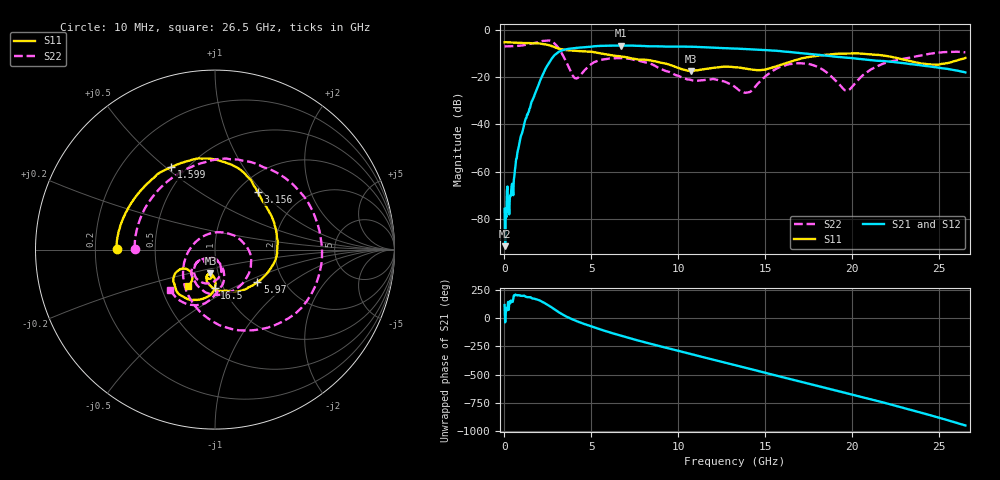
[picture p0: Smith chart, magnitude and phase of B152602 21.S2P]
!  2-Port S-parameters saved by WinCal
! VAR MeasName=S-Parameters (CALIBRATED_DATA) read from VNA (N5242A)
! VAR MeasDate=2016-1-5 16:28:22
! VAR NAME=B152602 21
! VAR FILENAME=B152602 21.S2P
! VAR DATE=2016-1-5 16:28:22
! VAR PHYS_PORTS=1,2
# Hz S DB R 50
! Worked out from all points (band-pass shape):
!   801 points, 10 MHz to 26.5 GHz, reference 50 ohm
!   highest |S21| = -6.62 dB at 6.699 GHz (marker M1); lowest = -91.6 dB at 43.11 MHz (marker M2)
!   |S21| within 3 dB of the highest: 3.062 GHz to 16.73 GHz (13.67 GHz wide, 138 % of centre)
!   lowest |S11| = -17.4 dB at 10.71 GHz (marker M3), VSWR 1.31, Z = 46 - j12.4 ohm
!   |S11| at or under -10 dB: 5.57 GHz to 19.66 GHz (14.09 GHz wide, 112 % of centre); 19.69 GHz to 19.82 GHz (129.6 MHz wide, 0.656 % of centre); 20.52 GHz to end of sweep
!   |S22| runs from -26.6 to -4.5 dB; largest |S21 - S12| = 0.0033
!   S11 on the Smith chart (normalised r, x): 10 MHz: 0.29, +0.00; 1.599 GHz: 0.41, +0.52; 3.156 GHz: 1.23, +0.94; 5.97 GHz: 1.48, -0.59; 16.5 GHz: 0.91, -0.41; 26.5 GHz: 0.68, -0.30
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1e7  -5.22 179.5  -75.76 114.6  -72.10 -24.6  -6.98 179.3
4.31125e7  -5.21 178.3  -91.58 -37.7  -91.47 168.6  -6.97 177.4
3.742375e8  -5.30 165.1  -70.14 154.6  -70.09 162.0  -6.92 157.0
8.70925e8  -5.50 146.3  -47.50 -159.8  -47.45 -158.1  -6.70 126.0
1.5994e9  -5.67 118.0  -29.98 173.9  -29.98 173.9  -5.71 75.6
2.460325e9  -6.30 80.3  -15.16 117.5  -15.17 117.5  -4.47 -4.4
2.824562e9  -7.11 64.5  -11.16 82.2  -11.16 82.2  -5.41 -51.7
3.155688e9  -7.98 53.3  -9.16 48.1  -9.16 48.1  -8.24 -95.2
3.9835e9  -8.78 28.2  -7.75 -16.8  -7.75 -16.7  -19.91 136.2
4.447075e9  -9.06 12.5  -7.45 -44.9  -7.45 -44.8  -18.56 48.3
5.97025e9  -10.53 -37.3  -6.67 -122.8  -6.66 -122.8  -12.16 -56.9
6.698725e9  -11.25 -55.5  -6.62 -155.9  -6.62 -155.9  -11.94 -84.6
8.851038e9  -13.64 -95.6  -6.93 114.9  -6.89 114.8  -16.02 -141.5
1.070534e10  -17.43 -100.8  -7.12 42.9  -7.10 42.9  -21.19 -139.2
1.3255e10  -15.82 -105.5  -7.90 -55.4  -7.88 -55.5  -24.15 -132.9
1.408281e10  -16.65 -106.3  -8.18 -87.6  -8.17 -87.6  -26.32 -92.6
1.650002e10  -13.33 -90.4  -9.44 177.7  -9.40 177.9  -14.39 -99.8
1.769208e10  -11.23 -101.4  -10.30 131.9  -10.25 132.0  -14.80 -128.5
1.967882e10  -10.00 -122.7  -11.77 56.5  -11.72 56.2  -25.74 -107.0
2.209604e10  -11.19 -146.6  -13.40 -38.0  -13.36 -38.2  -13.61 -80.4
2.46457e10  -14.68 -139.5  -15.65 -144.6  -15.65 -144.9  -9.88 -106.1
2.65e10  -11.89 -126.9  -18.00 132.4  -17.97 132.2  -9.51 -137.9
